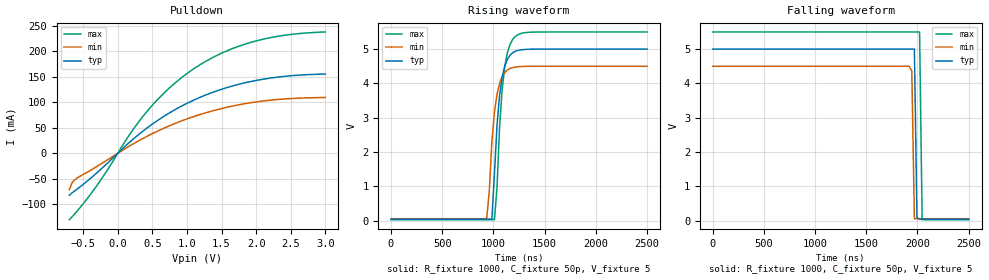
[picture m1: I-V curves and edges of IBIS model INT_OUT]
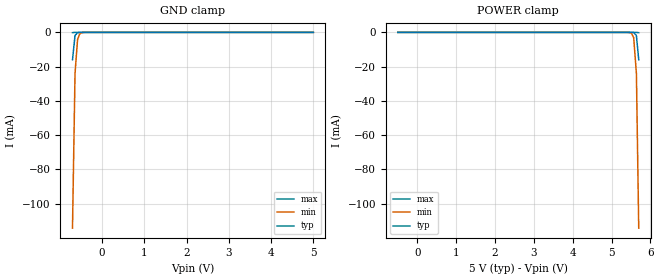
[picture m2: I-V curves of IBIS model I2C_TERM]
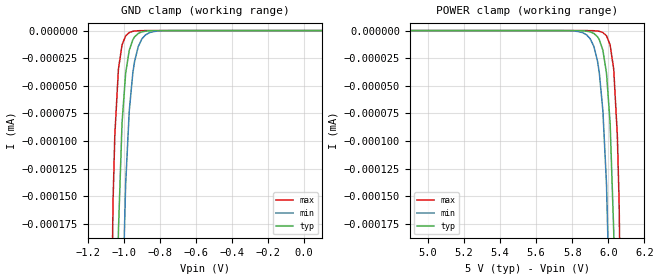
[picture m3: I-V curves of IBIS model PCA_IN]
|   NXP Semiconductors Inc.
|   Specialty Logic Products Group
|   IBIS model of PCA9544A
|   4-Channel I2C switch with
|   interrupt logic
[IBIS Ver]   3.2
[Comment Char]   |_char
| VDD typ = 5V, min = 4.5V and max = 5.5V
[File name]   pca9544a_5v.ibs
[File Rev]   1.0
[Date]   Nov 29, 2007 12:50:22 PM
[Source]
Generated by Seshadri Venkataramanan with IbisToolKit at Tempe, AZ
[Notes]
[Disclaimer]
* All rights reserved
NXP Semiconductors warrants and represents that the IBIS models identified
herein are owned by NXP Semiconductors (NXP). The
models provided are not warranted as fully representing all of the operating
characteristics and specifications of the semiconductor products to which the
models relate. Moreover, unless there is a
signed, written agreement to the contrary, these models are furnished on an "as
is" basis without support or warranty of any kind, either expressed or implied,
regarding the use thereof, and NXP specifically disclaims all implied warranties
of merchantability and
fitness of the models for any purpose.
NXP does not assume any liability arising out of the application or use of these
IBIS models including infringement of patents and
copyrights, nor does NXP convey any license under its patents and copyrights or
the rights of others.
NXP provides IBIS models as a service to our customers. You and your company
shall not distribute, convey, sell, or give these models
to anyone else without receiving prior written permission from NXP.(C) Copyright
2007 NXP Semiconductors
NXP Semiconductors (NXP) does not warrant that this model and any other
accompanying information (Model) accurately or fully represents the
operating characteristics and specifications of the semiconductor
products to which the Model relates.  Moreover, the Model is furnished
on an "as is" and with "all faults" basis, and without support or
warranty of any kind.  NXP disclaims all warranties, whether expressed
or implied or statutory, including without limitation all implied
warranties of non-infringement, merchantability and fitness for any
purpose, and those arising from a course of dealing or usage of trade.
NXP does not convey any license under its or any third party's patents,
copyrights or other intellectual property or proprietary rights.
You and your company assume any and all risks and liability arising out
of the application or use of the Model.
In no event shall NXP be liable for any direct, indirect, special,
consequential or incidental damages, however caused, whether in
warranty, contract or tort (including negligence), strict liability or
other legal theory, including, without limitation, for lost profits,
business interruption, or corruption or loss of data or information,
arising out of or in connection with the use of or the inability to use
the Model, even if NXP has been advised of the possibility of such
damages.
NXP provides the Model as a courtesy to our customers. You and your
company shall not distribute, convey, sell, or give the Model to anyone
else without receiving prior written permission from NXP.
NXP reserves the right to make changes without notice to the Model to
improve reliability, function, or design.
Please be aware that your receipt and subsequent use of the Model shall
serve as acceptance of these terms and conditions.  If you do not
accept these terms, return or destroy the Model immediately.
[Copyright]
2007
[Component]   PCA9544AD
Si_location Pin
Timing_location Pin
[Manufacturer]   NXP Semiconductors
[Package]
|   variable   typ   min   max
R_pkg   5.95E-02   5.36E-02   6.59E-02
L_pkg   4.21E-09   3.07E-09   5.91E-09
C_pkg   0.910E-12   0.758E-12   1.110E-12
|   SO20
[Pin] signal_name   model_name   R_pin   L_pin   C_pin
1   A0   PCA_IN   5.75E-02  5.91E-09  1.050E-12
2   A1   PCA_IN   6.25E-02  4.85E-09  1.040E-12
3   a2   PCA_IN   6.59E-02  3.92E-09  0.861E-12
4   INT0B   INT_IN   5.79E-02  3.32E-09  0.803E-12
5   SD0   I2C_TERM   5.36E-02  3.07E-09  0.758E-12
6   SC0   I2C_TERM   5.36E-02  3.07E-09  0.758E-12
7   INT1B   INT_IN   5.79E-02  3.32E-09  0.803E-12
8   SD1   I2C_TERM   6.59E-02  3.92E-09  0.861E-12
9   SC1   I2C_TERM   6.25E-02  4.85E-09  1.040E-12
10   Vss   GND   5.75E-02  5.91E-09  1.110E-12
11   INT2B   INT_IN   5.75E-02  5.91E-09  1.110E-12
12   SD2   I2C_TERM   6.25E-02  4.85E-09  1.040E-12
13   SC2   I2C_TERM   6.59E-02  3.92E-09  0.861E-12
14   INT3B   INT_IN   5.79E-02  3.32E-09  0.803E-12
15   SD3   I2C_TERM   5.36E-02  3.07E-09  0.758E-12
16   SC3   I2C_TERM   5.36E-02  3.07E-09  0.758E-12
17   INTB   INT_OUT   5.79E-02  3.32E-09  0.803E-12
18   SCL   I2C_TERM   6.59E-02  3.92E-09  0.861E-12
19   SDA   I2C_TERM   6.25E-02  4.85E-09  1.040E-12
20   Vdd   POWER   5.75E-02  5.91E-09  1.110E-12
[Series Pin Mapping] pin_2 model_name   function_table_group
18   6   PCA_SW   1
18   9   PCA_SW   2
18   13   PCA_SW   3
18   16   PCA_SW   4
19   5   PCA_SW   1
19   8   PCA_SW   2
19   12   PCA_SW   3
19   15   PCA_SW   4
[Series Switch Groups]
Off 1 2 3 4 /
On 1 /
On 2 /
On 3 /
On 4 /
[Component]   PCA9544APW
Si_location Pin
Timing_location Pin
[Manufacturer]   NXP Semiconductors
[Package]
|   variable   typ   min   max
R_pkg   7.24E-02   6.63E-02   8.34E-02
L_pkg   2.47E-09   2.09E-09   3.18E-09
C_pkg   0.341E-12   0.282E-12   0.420E-12
|   TSSOP20
[Pin] signal_name   model_name   R_pin   L_pin   C_pin
1   A0   PCA_IN   6.63E-02  3.18E-09  0.408E-12
2   A1   PCA_IN   6.67E-02  2.55E-09  0.398E-12
3   A2   PCA_IN   8.34E-02  2.35E-09  0.317E-12
4   INT0B   INT_IN   7.44E-02  2.16E-09  0.293E-12
5   SD0   I2C_TERM   7.10E-02  2.09E-09  0.282E-12
6   SC0   I2C_TERM   7.10E-02  2.09E-09  0.282E-12
7   INT1B   INT_IN   7.44E-02  2.16E-09  0.293E-12
8   SD1   I2C_TERM   8.34E-02  2.35E-09  0.317E-12
9   SC1   I2C_TERM   6.67E-02  2.55E-09  0.397E-12
10   Vss   GND   6.63E-02  3.18E-09  0.420E-12
11   INT2B   INT_IN   6.63E-02  3.17E-09  0.420E-12
12   SD2   I2C_TERM   6.67E-02  2.55E-09  0.397E-12
13   SC2   I2C_TERM   8.34E-02  2.35E-09  0.317E-12
14   INT3B   INT_IN   7.44E-02  2.16E-09  0.293E-12
15   SD3   I2C_TERM   7.10E-02  2.09E-09  0.282E-12
16   SC3   I2C_TERM   7.10E-02  2.09E-09  0.282E-12
17   INTB   INT_OUT   7.44E-02  2.16E-09  0.293E-12
18   SCL   I2C_TERM   8.34E-02  2.35E-09  0.317E-12
19   SDA   I2C_TERM   6.67E-02  2.55E-09  0.398E-12
20   Vdd   POWER   6.63E-02  3.17E-09  0.420E-12
[Series Pin Mapping] pin_2 model_name   function_table_group
16   3   PCA_SW   1
16   7   PCA_SW   2
16   11   PCA_SW   3
16   14   PCA_SW   4
17   3   PCA_SW   1
17   6   PCA_SW   2
17   10   PCA_SW   3
17   13   PCA_SW   4
[Series Switch Groups]
Off 1 2 3 4 /
On 1 /
On 2 /
On 3 /
On 4 /
[Component]   PCA9544ABS
Si_location Pin
Timing_location Pin
[Manufacturer]   NXP Semiconductors
[Package]
|   variable   typ   min   max
R_pkg   0.364   0.215   0.513
L_pkg   1.49E-09   1.04E-09   1.93E-09
C_pkg   0.149E-12   0.124E-12   0.173E-12
|   HVQFN20
[Package Model]   hvqfn20
[Pin] signal_name   model_name
1   A2   PCA_IN
2   INT0B   INT_IN
3   SD0   I2C_TERM
4   SC0   I2C_TERM
5   INT1B   INT_IN
6   SD1   I2C_TERM
7   SC1   I2C_TERM
8   Vss   GND
9   INT2B   INT_IN
10   SD2   I2C_TERM
11   SC2   I2C_TERM
12   INT3B   INT_IN
13   SD3   I2C_TERM
14   SC3   I2C_TERM
15   INTB   INT_OUT
16   SCL   I2C_TERM
17   SDA   I2C_TERM
18   Vdd   POWER
19   A0   PCA_IN
20   A1   PCA_IN
[Series Pin Mapping] pin_2 model_name   function_table_group
18   6   PCA_SW   1
18   9   PCA_SW   2
18   13   PCA_SW   3
18   16   PCA_SW   4
19   5   PCA_SW   1
19   8   PCA_SW   2
19   12   PCA_SW   3
19   15   PCA_SW   4
[Series Switch Groups]
|   Function Group States
|  default
Off 1 2 3 4 /
On 1 /
On 2 /
On 3 /
On 4 /
|  [Define Package Model]  MLF20_PCA9564.pkg
[Define Package Model]   hvqfn20
[Manufacturer]   Unknown
[OEM]   Unknown
[Description]   none
[Number of Pins]   20
[Pin Numbers]
|   1 = D2
1
|   2 = D3
2
|   3 = D4
3
|   4 = D5
4
|   5 = D6
5
|   6 = D7
6
|   7 = NC
7
|   8 = Vss
8
|   9 = WRn
9
|   10 = RDn
10
|   11 = CEn
11
|   12 = A0
12
|   13 = A1
13
|   14 = INTn
14
|   15 = RESETn
15
|   16 = SCL
16
|   17 = SDA
17
|   18 = Vdd
18
|   19 = D0
19
|   20 = D1
20
[Model Data]
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[End Model Data]
[End Package Model]
[Model]   PCA_SW
Model_type Series_switch
C_comp   0   0   0
[Temperature Range] 27   85   -40
[Voltage Range]   5   4.5   5.5
[On]
[R Series]   9   4   24
[C Series]   3p   2p   5p
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[Off]
|   variable   R(typ)   R(min)   R(max)
[R Series]   1e07   1e07   1e07
[L Series]   0   0   0
[C Series]   0   0   0
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| Models and submodels in the file (5): INT_OUT (Open_drain), I2C_TERM (Terminator), PCA_IN (Input), INT_IN (Input), PCA_SW (Series_switch)
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[Model]   INT_OUT
Model_type Open_drain
Vref=5
Vmeas=1.25
Rref=1000
Cref=1p
C_comp   2.2p   2p   2.3p
[Model Spec]
Vmeas   2.5   2.25   2.75
[Temperature Range] 27   85   -40
[Voltage Range]   5   4.5   5.5
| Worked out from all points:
|   slope of the pulldown table from 0 to 0.75 V, typ, clamps not added: 9.44 ohm
|   falling waveform, R_fixture 1000, C_fixture 50p, V_fixture 5: 20-80 % time 15.3ns typ, 15.6ns min, 15.2ns max; typ from 5 V to 0.038 V
|   rising waveform, R_fixture 1000, C_fixture 50p, V_fixture 5: 20-80 % time 73.3ns typ, 70.6ns min, 70.2ns max; typ from 0.038 V to 5 V
[Pulldown]
-700mV    -82.55mA   -71.37mA   -130.3mA
-660mV    -77.67mA   -57.63mA   -124.6mA
-590mV    -70.48mA   -48.78mA   -113.9mA
-290mV    -36.9mA    -24.88mA   -61.08mA
160mV     20.36mA    13.43mA    34.43mA
380mV     45.19mA    30.2mA     75.04mA
680mV     73.62mA    49.98mA    119.7mA
980mV     96.57mA    66.43mA    154.4mA
1.39V     120.4mA    83.97mA    189.1mA
1.88V     139.5mA    98.23mA    215.8mA
2.4V      150.8mA    106.4mA    231.3mA
3V        155.5mA    109.4mA    238mA
[Falling Waveform]
R_fixture=1000
C_fixture=50p
V_fixture=5
V_fixture_min=4.5
V_fixture_max=5.5
0s        5V         4.5V       5.5V
1.919us   5V         4.5V       5.5V
1.944us   5V         4.361V     5.5V
1.97us    5V         52.07mV    5.5V
1.995us   86.07mV    51.74mV    5.5V
2.02us    37.66mV    51.74mV    5.5V
2.045us   37.66mV    51.74mV    30.18mV
2.5us     37.66mV    51.74mV    24.21mV
[Rising Waveform]
R_fixture=1000
C_fixture=50p
V_fixture=5
V_fixture_min=4.5
V_fixture_max=5.5
0s        37.66mV    51.74mV    24.19mV
934.3ns   37.7mV     51.77mV    24.26mV
984.8ns   37.75mV    2.289V     24.27mV
1.01us    1.361V     3.159V     24.3mV
1.035us   2.794V     3.687V     968.5mV
1.061us   3.663V     4.007V     2.754V
1.086us   4.19V      4.201V     3.837V
1.136us   4.703V     4.39V      4.89V
1.212us   4.934V     4.476V     5.365V
2.5us     5V         4.5V       5.5V
[Ramp]
R_load=1000
dV/dt_r   2.977E+0/1.073E-9   2.965E+0/1.246E-9   2.987E+0/1.228E-9
dV/dt_f   2.977E+0/7.078E-10   2.965E+0/1.185E-9   2.987E+0/6.063E-10
|[End   INT_OUT
| [End   INT_OUT
|  [End   INT_OUT
[Model]   I2C_TERM
Model_type Terminator
C_comp   1.7p   1.7p   1.7p
[Temperature Range] 27   85   -40
[Voltage Range]   5   4.5   5.5
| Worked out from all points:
|   GND clamp passes 1 mA (typ) near -0.61 V on its own axis
[GND Clamp]
|   -6.000000E-1   -1.554225E-1   -1.242642E-1   -2.666059E-1
|   -5.000000E-1   -1.602113E-1   -1.179351E-1   -2.662641E-1
|   -4.000000E-1   -1.574088E-1   -1.099432E-1   -2.800035E-1
-700mV    -15.98mA   -114.2mA   -166.1uA
-640mV    -1.824mA   -23.99mA   -8.398uA
-580mV    -183.2uA   -4.199mA   -424nA
-530mV    -26.56uA   -872.2uA   -35.29nA
-470mV    -2.612uA   -126.3uA   -1.868nA
-350mV    -25.3nA    -2.592uA   -73.47pA
5V        893.1pA    979.7pA    937.7pA
[POWER Clamp]
-500mV    942.7pA    1.037nA    987.3pA
5.32V     -7.973nA   -980.6nA   -64.06pA
5.51V     -12.26uA   -459.2uA   -13.1nA
5.57V     -124.5uA   -3.085mA   -257.8nA
5.64V     -1.824mA   -23.99mA   -8.398uA
5.7V      -15.98mA   -114.2mA   -166.1uA
[Model]   PCA_IN
Model_type Input
Vinh=2.1
Vinl=0.9
C_comp   0.5p   0.5p   0.5p
[Model Spec]
[Temperature Range] 27   85   -40
[Voltage Range]   5   4.5   5.5
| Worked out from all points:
|   GND clamp passes 1 mA (typ) near -1.25 V on its own axis
[GND Clamp]
-1.7V     -4.583A    -3.655A    -5.795A
-1.08V    -1.254uA   -2.572uA   -421.3nA
-1.06V    -578.9nA   -1.345uA   -155.7nA
-1.05V    -393.3nA   -972.8nA   -94.64nA
-1.03V    -181.5nA   -508.9nA   -34.97nA
-1.01V    -83.76nA   -266.2nA   -12.93nA
-990mV    -38.66nA   -139.2nA   -4.777nA
-970mV    -17.84nA   -72.82nA   -1.766nA
-950mV    -8.234nA   -38.09nA   -653.2pA
-920mV    -2.582nA   -14.41nA   -147.4pA
-860mV    -254.6pA   -2.063nA   -8.255pA
100mV     100fA      100fA      100fA
[POWER Clamp]
4.9V      100fA      100fA      100fA
5.86V     -254.6pA   -2.063nA   -8.255pA
5.92V     -2.582nA   -14.41nA   -147.4pA
5.95V     -8.234nA   -38.09nA   -653.2pA
5.97V     -17.84nA   -72.82nA   -1.766nA
5.99V     -38.66nA   -139.2nA   -4.777nA
6.01V     -83.76nA   -266.2nA   -12.93nA
6.03V     -181.5nA   -508.9nA   -34.97nA
6.05V     -393.3nA   -972.8nA   -94.64nA
6.06V     -578.9nA   -1.345uA   -155.7nA
6.08V     -1.254uA   -2.572uA   -421.3nA
6.7V      -4.583A    -3.655A    -5.795A
